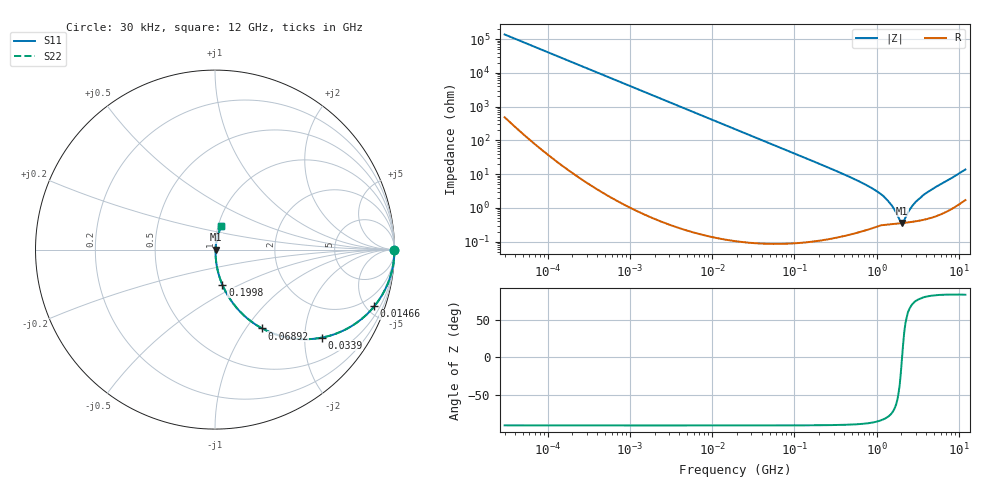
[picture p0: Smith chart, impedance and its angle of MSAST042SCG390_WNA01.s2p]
! MSAST042SCG390_WNA01  S-PARAMETER MODEL  ( General Type )
! Model Generated by TAIYO YUDEN Corporation (http://www.ty-top.com)
! Version 1.0
! TAIYO YUDEN Control No. 150820
! Copyright(c) 2015 TAIYO YUDEN CO.,LTD. All Rights Reserved.
! Product Description (link to TY-COMPAS)
! https://ds.yuden.co.jp/TYCOMPAS/or/detail?pn=MSAST042SCG390JWNA01&u=M
! Products Name : Multilayer Ceramic Capacitors
! Characteristics :
!  Capacitance : 39 pF , Rated Voltage : 25V , TCC : CG / C0G
!  Case Size : 0.4 x 0.2 / 0.016 x 0.008 [mm/inch] , Thickness : 0.2 / 0.008 [mm/inch]
!  (Conditions: Temperature = 25 degC , DC Bias Current/Voltage = 0A / 0V)
! External Node Assignments :
!  1  o---| |---o  2
! GND o---------o GND
! Frequency Range : 0.03MHz  -  12000MHz  [ 401 STEP ]
# MHz S RI R 50
! Freq[MHz].  S11 Real  S11 Imag  S21 Real  S21 Imag  S12 Real  S12 Imag  S22 Real  S22 Imag
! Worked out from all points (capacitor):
!   401 points, 30 kHz to 12 GHz, reference 50 ohm
!   read as one part in series: C = 38.7 pF near 32 kHz
!   lowest |Z| = 355 mohm at 2.037 GHz (marker M1)
!   series resonance near 2.038 GHz, so ESL is about 160 pH
!   S11 on the Smith chart (normalised r, x): 30 kHz: open; 14.66 MHz: 1.00, -5.61; 33.9 MHz: 1.00, -2.43; 68.92 MHz: 1.00, -1.19; 199.8 MHz: 1.00, -0.41; 12 GHz: 1.03, +0.27
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0.03  1 -0.000729  3.11e-06 0.000729  3.11e-06 0.000729  1 -0.000729
0.260295  1 -0.00633  4.28e-05 0.00633  4.28e-05 0.00633  1 -0.00633
2.258455  0.997 -0.0547  0.00302 0.0547  0.00302 0.0547  0.997 -0.0547
6.13721  0.9782 -0.1459  0.0218 0.1459  0.0218 0.1459  0.9782 -0.1459
14.65919  0.8872 -0.3161  0.1128 0.3161  0.1128 0.3161  0.8872 -0.3161
18.97367  0.8245 -0.3802  0.1755 0.3802  0.1755 0.3802  0.8245 -0.3802
33.90345  0.5953 -0.4905  0.4047 0.4905  0.4047 0.4905  0.5953 -0.4905
68.9219  0.2626 -0.4393  0.7374 0.4393  0.7374 0.4393  0.2626 -0.4393
104.8152  0.1335 -0.3389  0.8665 0.3389  0.8665 0.3389  0.1335 -0.3389
164.6252  0.0589 -0.2334  0.9411 0.2334  0.9411 0.2334  0.0589 -0.2334
199.7686  0.0409 -0.1954  0.9591 0.1954  0.9591 0.1954  0.0409 -0.1954
774.0045  0.00431 -0.0453  0.9957 0.0453  0.9957 0.0453  0.00431 -0.0453
1139.739  0.00368 -0.0248  0.9963 0.0248  0.9963 0.0248  0.00368 -0.0248
1428.372  0.00344 -0.014  0.9966 0.014  0.9966 0.014  0.00344 -0.014
1625.032  0.00342 -0.00878  0.9966 0.00878  0.9966 0.00878  0.00342 -0.00878
1909.359  0.00349 -0.00252  0.9965 0.00252  0.9965 0.00252  0.00349 -0.00252
2036.564  0.00354 -3.37e-05  0.9965 3.37e-05  0.9965 3.37e-05  0.00354 -3.37e-05
2172.242  0.00361 0.00247  0.9964 -0.00247  0.9964 -0.00247  0.00361 0.00247
2552.314  0.00385 0.0084  0.9962 -0.0084  0.9962 -0.0084  0.00385 0.0084
2811.574  0.00405 0.012  0.996 -0.012  0.996 -0.012  0.00405 0.012
3758.338  0.00503 0.0241  0.995 -0.0241  0.995 -0.0241  0.00503 0.0241
12000  0.0341 0.1292  0.9659 -0.1292  0.9659 -0.1292  0.0341 0.1292
